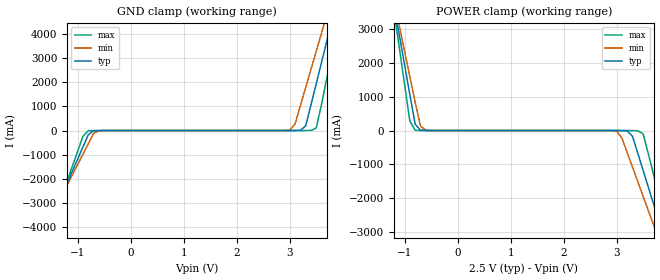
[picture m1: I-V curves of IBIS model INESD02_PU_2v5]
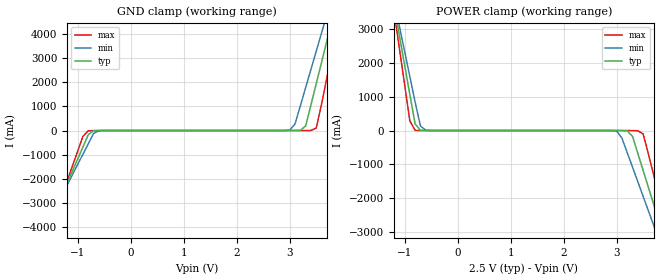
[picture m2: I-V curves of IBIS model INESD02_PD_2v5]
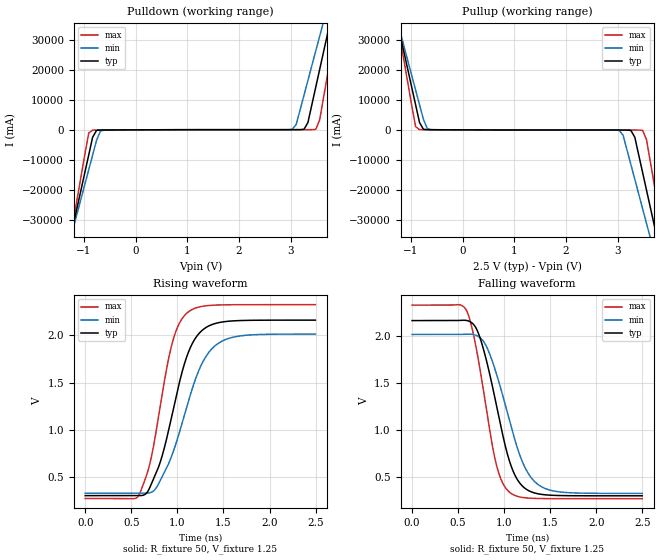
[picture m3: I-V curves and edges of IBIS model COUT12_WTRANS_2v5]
|   This file is an IBIS representation of the   |
|   Integrated Device Technology,Inc.   |
|   ICS840004I-01   |
|   XTAL to  LVCMOS/LVTTL Frequency Synthesizer   |
[IBIS Ver]   4.1
[File name]   840004i_01.ibs
[File Rev]   1.0
[Date]   15 Jun 2009 | Last modified
|   Sep 27 2007 | Generated
[Source]   Originated at Integrated Devices Technology, Inc.
[Disclaimer]
IDT hereby grants the user of this IBIS model a non-exclusive,
nontransferable license to use this IBIS model under the following terms.
Before using this IBIS model, the user should read this license.
If the user does not accept these terms,  the IBIS model should be
returned to IDT within 30 days.
   The user is granted this license only to use the IBIS model and
is not granted rights to sell, load, rent, lease or license the IBIS
model in whole or in part, or in modified form to anyone other than
user. User may modify the IBIS model to suit its specific
applications but rights to derivative works and such modifications
shall belong to IDT.
   This IBIS model is provided on an "AS IS" basis and IDT makes
absolutely no warranty with respect to the information contained
herein. IDT DISCLAIMS AND CUSTOMER WAIVES ALL WARRANTIES, EXPRESS
OR IMPLIED, INCLUDING WARRANTIES OF MERCHANTABILITY OR FITNESS FOR
A PARTICULAR PURPOSE. The entire risk as to quality and performance
is with the Customer. ACCORDINGLY, IN NO EVENT SHALL THE COMPANY BE
LIABLE FOR ANY DAMAGES, WHETHER IN CONTRACT OR TORT,INCLUDING ANY
LOST PROFITS OR OTHER INCIDENTAL, CONSEQUENTIAL, EXEMPLARY, OR
PUNITIVE DAMAGES ARISING OUT OF THE USE OR APPLICATION OF THE IBIS
model provided in this package. Further, IDT reserves the right to
make changes without notice to any product herein to improve
reliability, function, or design. IDT does not convey any license
under patent rights or any other intellectual property rights,
including those of third parties.
   IDT is not obligated to provide maintenance or support
for the licensed IBIS model.
[Copyright]   Copyright 2007 by Integrated Device Technology,Inc
[Component]   ICS840004GI-01
[Manufacturer] Integrated Devices Technology, Inc.
[Package]
|TSSOP 20 Lead
|   typ   min   max
R_pkg   51.85m   41.1m   62.6m
L_pkg   1.568nH   0.734nH   2.401nH
C_pkg   0.221pF   0.068pF   0.373pF
[Pin] signal_name  model_name   R_pin   L_pin   C_pin
1   F_SEL0   INESD02_PU   62.6m   2.401n   0.373p
2   NC   NC   57.23m   1.985n   0.297p
3   nXTAL_SEL   INESD02_PD   51.85m   1.568n   0.221p
4   REF_CLK   INESD02_PD   46.78m   1.151n   0.145p
5   OE   INESD02_PU   41.1m   0.734n   0.068p
6   MR   INESD02_PD   41.1m   0.734n   0.068p
7   nPLL_SEL   INESD02_PD   46.78m   1.151n   0.145p
8   VDDA   POWER   51.85m   1.568n   0.221p
9   NC   NC   57.23m   1.985n   0.297p
10   VDD   POWER   62.6m   2.401n   0.373p
11   XTAL_OUT   NC   62.6m   2.401n   0.373p
12   XTAL_IN   NC   57.23m   1.985n   0.297p
13   GND   GND   51.85m   1.568n   0.221p
14   Q3   COUT12_WTRANS  46.78m   1.151n   0.145p
15   Q2   COUT12_WTRANS  41.1m   0.734n   0.068p
16   VDDO   POWER   41.1m   0.734n   0.068p
17   Q1   COUT12_WTRANS  46.78m   1.151n   0.145p
18   Q0   COUT12_WTRANS  51.85m   1.568n   0.221p
19   GND   GND   57.23m   1.985n   0.297p
20   F_SEL1   INESD02_PU   62.6m   2.401n   0.373p
[Model Selector] INESD02_PU
INESD02_PU_2v5  Buffer selection for 2v5
INESD02_PU_3v3  Buffer selection for 3v3
[Model Selector] INESD02_PD
INESD02_PD_2v5  Buffer selection for 2v5
INESD02_PD_3v3  Buffer selection for 3v3
[Model Selector] COUT12_WTRANS
COUT12_WTRANS_2v5  Buffer selection for 2v5
COUT12_WTRANS_3v3  Buffer selection for 3v3
| Models and submodels in the file (6): INESD02_PU_2v5 (Input), INESD02_PD_2v5 (Input), COUT12_WTRANS_2v5 (Output), INESD02_PU_3v3 (Input), INESD02_PD_3v3 (Input), COUT12_WTRANS_3v3 (Output)
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[Model] INESD02_PU_2v5
Model_type   Input
Polarity   Non-Inverting
Vinl = 1.4V
Vinh = 1.85V
|   typ   min   max
C_comp   2pF   1.5pF   2.5pF
|   typ   min   max
[Voltage range]  2.5V   2.375V   2.625V
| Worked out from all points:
|   GND clamp passes 1 mA (typ) near -0.55 V on its own axis
|   POWER clamp passes 1 mA (typ) near -0.61 V on its own axis
[GND_clamp]
|Voltage   I(typ)   I(min)   I(max)
-2.5V     -8.775A    -7.892A    -10.18A
-1.6V     -4.218A    -4.001A    -4.586A
-900mV    -678.5mA   -979.4mA   -237.6mA
-800mV    -173.9mA   -548.7mA   -10.88mA
-600mV    -1.682mA   -8.796mA   -960.5uA
3V        79.39uA    17.1mA     7.198uA
3.1V      607uA      273.4mA    11.46uA
3.3V      191.5mA    1.785A     278.5uA
3.5V      1.949A     3.298A     103.5mA
3.7V      3.723A     4.812A     2.189A
3.9V      5.498A     6.327A     4.369A
5V        15.27A     14.67A     16.38A
[POWER_clamp]
|Voltage   I(typ)   I(min)   I(max)
-2.5V     15.27A     13.72A     17.74A
-1.2V     3.723A     3.866A     3.551A
-1.1V     2.836A     3.109A     2.461A
-900mV    1.063A     1.596A     283.3mA
-800mV    191.5mA    840mA      6.139mA
-600mV    607uA      8.789mA    64.82uA
3V        -392uA     -16.42mA   -62.09uA
3.4V      -678.5mA   -1.518A    -7.233mA
3.5V      -1.184A    -1.95A     -99.57mA
3.7V      -2.195A    -2.813A    -1.324A
4V        -3.712A    -4.109A    -3.188A
5V        -8.775A    -8.433A    -9.404A
[Model] INESD02_PD_2v5
Model_type   Input
Polarity   Non-Inverting
Vinl = 1.4V
Vinh = 1.85V
|   typ   min   max
C_comp   2pF   1.5pF   2.5pF
|   typ   min   max
[Voltage range]  2.5V   2.375V   2.625V
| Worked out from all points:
|   GND clamp passes 1 mA (typ) near -0.55 V on its own axis
|   POWER clamp passes 1 mA (typ) near -0.60 V on its own axis
[GND_clamp]
|Voltage I(typ)   I(min)   I(max)
-2.5V     -8.775A    -7.892A    -10.18A
-1.6V     -4.218A    -4.001A    -4.586A
-900mV    -678.5mA   -979.3mA   -237.6mA
-800mV    -173.9mA   -548.7mA   -10.83mA
-600mV    -1.629mA   -8.74mA    -911.1uA
3V        133.3uA    17.16mA    56.6uA
3.1V      660.9uA    273.5mA    60.87uA
3.3V      191.6mA    1.785A     327.9uA
3.5V      1.949A     3.298A     103.6mA
3.7V      3.723A     4.812A     2.189A
3.9V      5.498A     6.327A     4.369A
5V        15.27A     14.67A     16.38A
[POWER_clamp]
|Voltage   I(typ)   I(min)   I(max)
-2.5V     15.27A     13.72A     17.74A
-1.2V     3.723A     3.866A     3.551A
-1.1V     2.836A     3.109A     2.461A
-900mV    1.063A     1.596A     283.3mA
-800mV    191.6mA    840.1mA    6.189mA
-600mV    660.9uA    8.845mA    114.2uA
3V        -338.1uA   -16.36mA   -12.68uA
3.4V      -678.5mA   -1.518A    -7.183mA
3.5V      -1.183A    -1.95A     -99.52mA
3.7V      -2.195A    -2.813A    -1.324A
4V        -3.712A    -4.109A    -3.188A
5V        -8.775A    -8.432A    -9.404A
[Model] COUT12_WTRANS_2v5
Model_type   Output
Polarity   Non-Inverting
|   typ   min   max
C_comp   2pF   1.5pF   2.5pF
Vmeas = 1.25V
Rref = 50
Cref = 50
Vref = 1.25V
|   typ   min   max
[Voltage range]   2.5V   2.375V   2.625V
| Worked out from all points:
|   slope of the pulldown table from 0 to 0.375 V, typ, clamps not added: 16.5 ohm
|   slope of the pullup table from 0 to 0.375 V, typ, clamps not added: 18.9 ohm
|   rising waveform, R_fixture 50, V_fixture 1.25: 20-80 % time 288ps typ, 340ps min, 232ps max; typ from 0.303 V to 2.16 V
|   falling waveform, R_fixture 50, V_fixture 1.25: 20-80 % time 262ps typ, 307ps min, 215ps max; typ from 2.16 V to 0.303 V
[Pulldown]
|Voltage   I (typ)   I (min)   I (max)
-2.5V     -132.4A    -116.6A    -159.3A
-1.288V   -37.91A    -37.91A    -38.44A
-1.212V   -32A       -32.99A    -30.89A
-909.1mV  -8.368A    -13.32A    -1.073A
-833.3mV  -2.461A    -8.397A    -92.21mA
-606.1mV  -40.23mA   -65.84mA   -45.64mA
3.03V     52.18mA    193.7mA    61.66mA
3.333V    2.453A     16.49A     62.14mA
3.485V    14.25A     26.32A     148.7mA
3.712V    31.96A     41.06A     18.39A
3.864V    43.76A     50.89A     33.49A
5V        132.3A     124.6A     146.7A
[Pullup]
|Voltage   I (typ)   I (min)   I (max)
-2.5V     132.4A     116.6A     159.3A
-1.288V   37.88A     37.89A     38.42A
-1.212V   31.98A     32.97A     30.87A
-909.1mV  8.357A     13.31A     1.064A
-833.3mV  2.454A     8.39A      87.48mA
-606.1mV  38.86mA    63.99mA    46.61mA
3.03V     -57.97mA   -201.8mA   -71.64mA
3.333V    -2.473A    -16.52A    -77.44mA
3.485V    -14.28A    -26.35A    -176.1mA
3.712V    -32A       -41.11A    -18.44A
3.864V    -43.82A    -50.94A    -33.55A
5V        -132.4A    -124.7A    -146.8A
[Ramp]
|   typ   min   max
dV/dt_r   1.486/0.453n   1.348/0.531n   1.642/0.366n
dV/dt_f   1.489/0.396n   1.35/0.466n   1.645/0.325n
R_load =   50.0000
[Rising Waveform]
R_fixture = 50
V_fixture = 1.25   |Vcc_typ
V_fixture_min = 1.1875 |Vcc_min
V_fixture_max = 1.3125 |Vcc_max
C_fixture = 0.0p
| Time   typ   min   max
0s        302.6mV    327.8mV    272.2mV
583.1ps   301.6mV    328mV      307.8mV
700.7ps   387.7mV    332.6mV    637.8mV
805.8ps   632.8mV    446.5mV    1.199V
951ps     1.196V     756mV      1.941V
1.021ns   1.496V     968.5mV    2.126V
1.109ns   1.791V     1.264V     2.239V
1.279ns   2.06V      1.723V     2.308V
1.474ns   2.139V     1.933V     2.322V
2.498ns   2.16V      2.013V     2.324V
[Falling Waveform]
R_fixture = 50
V_fixture = 1.25   |Vcc_typ
V_fixture_min = 1.1875 |Vcc_min
V_fixture_max = 1.3125 |Vcc_max
C_fixture = 0.0p
| Time   typ   min   max
0s        2.16V      2.013V     2.324V
590.6ps   2.162V     2.016V     2.267V
653.2ps   2.133V     2.014V     2.069V
728.2ps   2.003V     1.986V     1.696V
908.4ps   1.296V     1.617V     657.8mV
976ps     982.4mV    1.393V     452.7mV
1.059ns   665.1mV    1.096V     339.6mV
1.224ns   383.1mV    606mV      281.8mV
1.406ns   317.5mV    397.7mV    273.6mV
2.498ns   302.6mV    327.8mV    272.2mV
